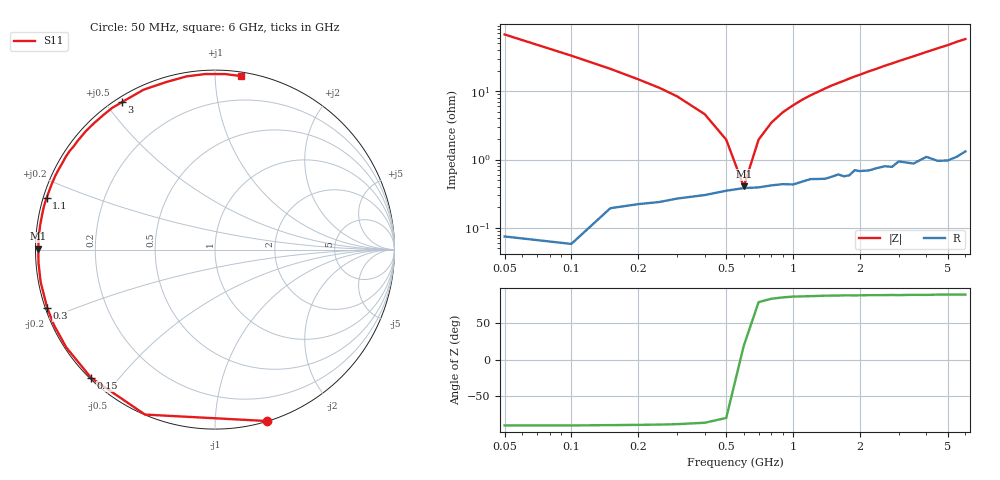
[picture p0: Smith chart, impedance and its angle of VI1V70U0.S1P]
! Infineon Technologies  Discrete & RF Semiconductors
! BB 804
! Si Tuning Diode in SOT23
! VR = 1.75 V
! S-Parameters:  July  1999
# GHz  S  MA  R  50
!  f  S11
! GHz  MAG  ANG
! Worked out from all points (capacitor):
!   34 points, 50 MHz to 6 GHz, reference 50 ohm
!   read as one part to ground: C = 46.8 pF near 50 MHz
!   lowest |Z| = 404 mohm at 600 MHz (marker M1)
!   series resonance near 593.6 MHz, so ESL is about 1.5 nH
!   S11 on the Smith chart (normalised r, x): 50 MHz: 0.00, -1.35; 150 MHz: 0.00, -0.42; 300 MHz: 0.01, -0.17; 1.1 GHz: 0.01, +0.15; 3 GHz: 0.02, +0.55; 6 GHz: 0.03, +1.16
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0.05  0.9989 -73.0
0.1  0.9984 -113.0
0.15  0.9934 -134.0
0.2  0.9919 -146.7
0.25  0.9909 -154.8
0.3  0.9896 -160.9
0.4  0.9881 -169.5
0.5  0.9861 -175.6
0.6  0.9848 179.7
0.7  0.9845 175.6
0.8  0.9835 172.1
0.9  0.9828 168.8
1.1  0.9816 163.0
1.4  0.9802 155.2
1.6  0.9776 150.5
1.7  0.9792 148.3
1.9  0.975 143.7
2.2  0.9762 137.4
2.4  0.9749 133.6
2.6  0.9742 129.5
2.8  0.9755 126.0
3  0.9716 122.3
3.5  0.9757 114.1
4  0.9724 106.3
4.5  0.978 99.3
5  0.9797 93.2
5.5  0.9794 86.7
6  0.9777 81.6
